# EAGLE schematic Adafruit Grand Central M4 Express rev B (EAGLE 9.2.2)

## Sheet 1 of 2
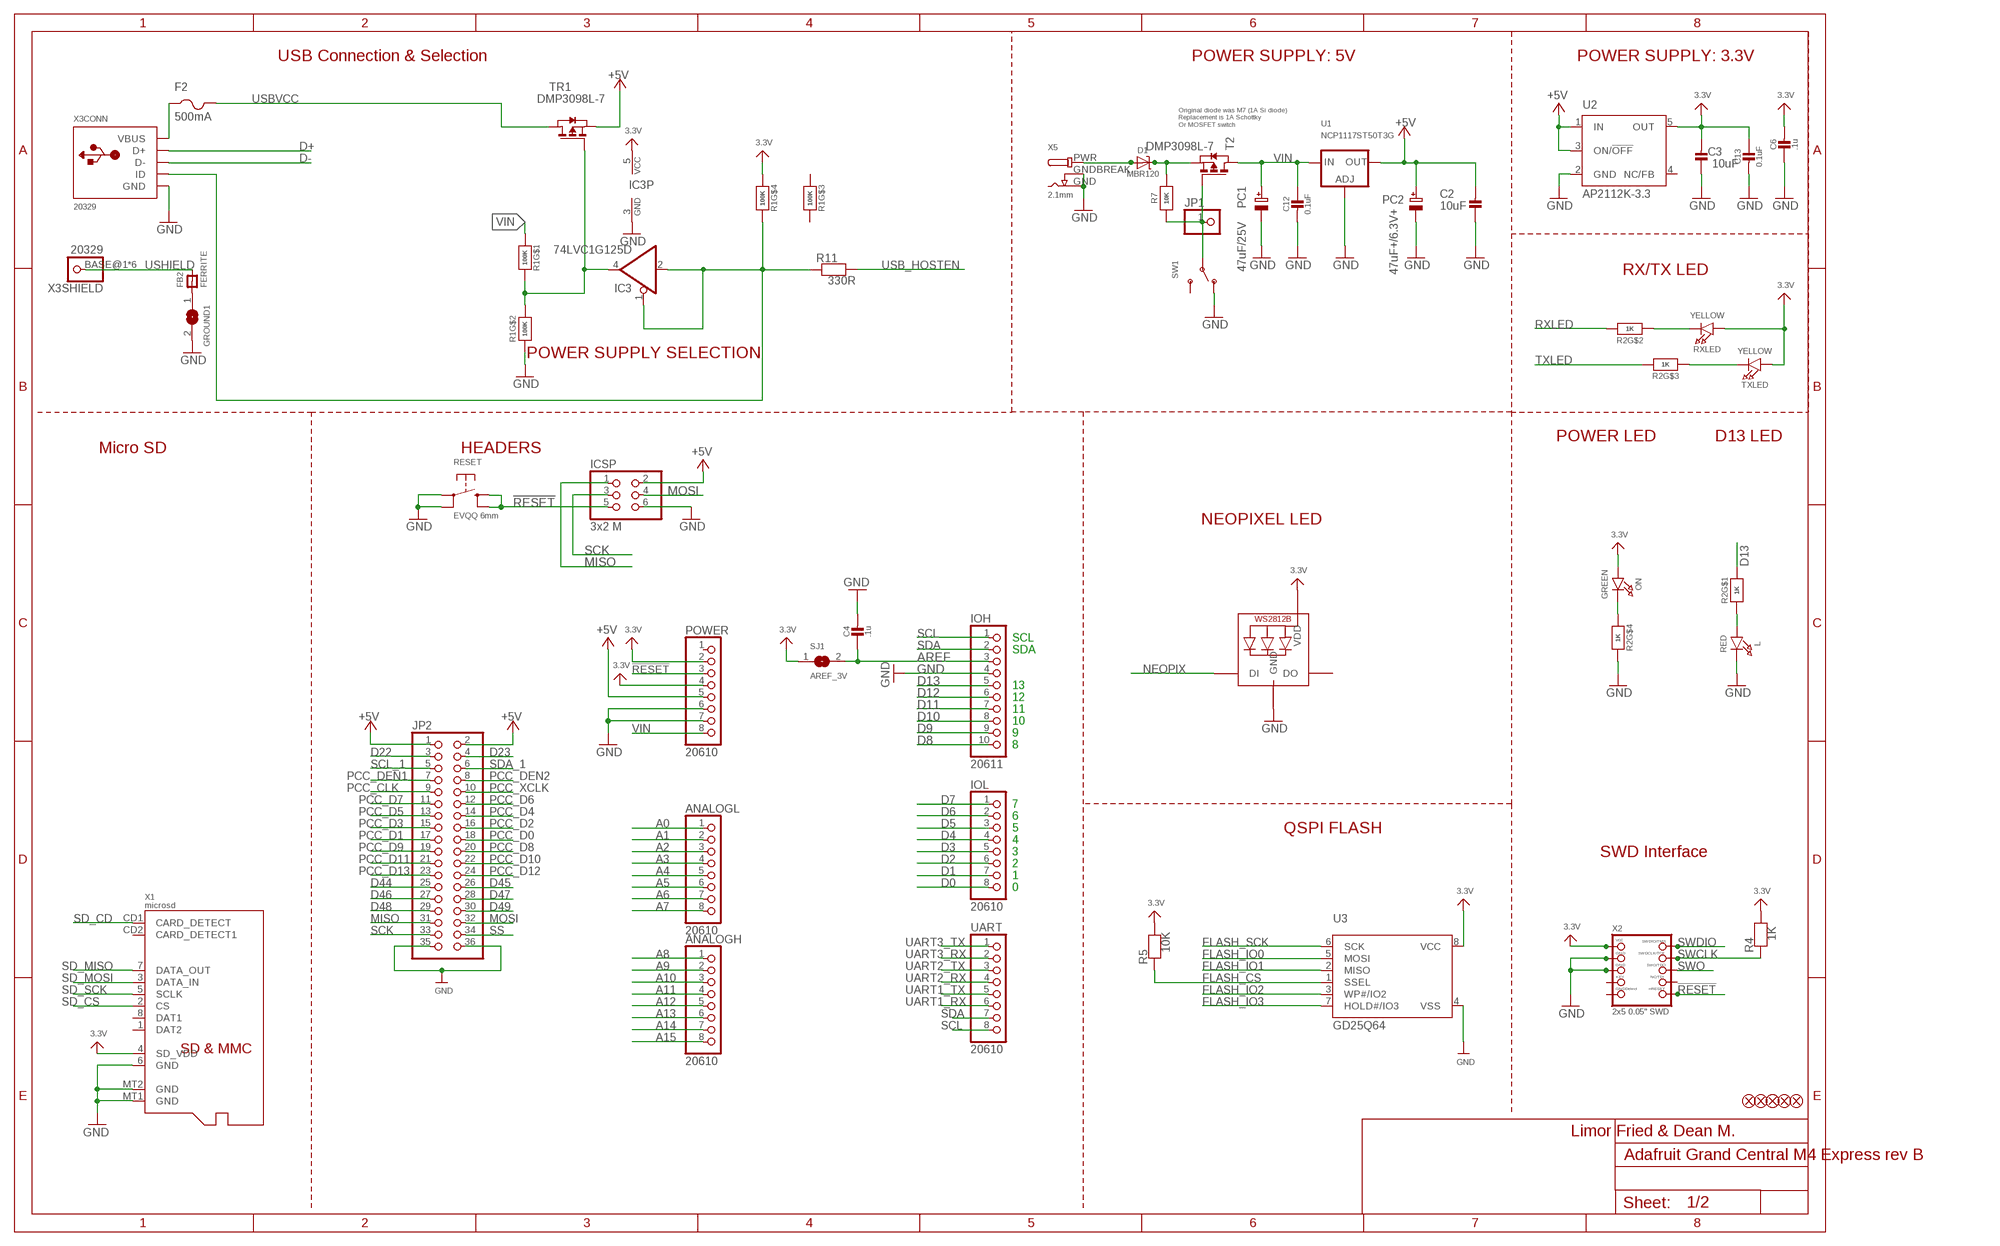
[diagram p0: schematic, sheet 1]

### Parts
ANALOGH  20610  HEADER-1X8OVALWAVE  [1X08_OVALWAVE]
ANALOGL  20610  HEADER-1X8OVALWAVE  [1X08_OVALWAVE]
C2  10uF  CAP_CERAMIC0805-NOOUTLINE  [0805-NO]
C3  10uF  CAP_CERAMIC0805-NOOUTLINE  [0805-NO]
C4  .1u  CAP_CERAMIC0603_NO  [0603-NO]
C6  .1u  CAP_CERAMIC0603_NO  [0603-NO]
C12  0.1uF  CAP_CERAMIC0603_NO  [0603-NO]
C13  0.1uF  CAP_CERAMIC0603_NO  [0603-NO]
D1  MBR120  DIODE-SCHOTTKYSOD-123  [SOD-123]
F2  500mA  PTCFUSE-1206  [R1206]
FB2  FERRITE  FERRITE-0805NO  [0805-NO]
FD1  FIDUCIAL_1MM  [FIDUCIAL_1MM]
FD2  FIDUCIAL_1MM  [FIDUCIAL_1MM]
FD3  FIDUCIAL_1MM  [FIDUCIAL_1MM]
FD4  FIDUCIAL_1MM  [FIDUCIAL_1MM]
FD5  FIDUCIAL_1MM  [FIDUCIAL_1MM]
GROUND1  SOLDERJUMPERCLOSED  [SOLDERJUMPER_CLOSEDWIRE]
IC3  74LVC1G125D  74AHC1G125DBV  [SOT23-5]
ICSP  3x2 M  HEADER-2X3  [2X03_ROUND_70MIL]
IOH  20611  HEADER-1X10OVALWAVE  [1X10_OVALWAVE]
IOL  20610  HEADER-1X8OVALWAVE  [1X08_OVALWAVE]
JP1  HEADER-1X1ROUND  [1X01_ROUND]
JP2  PINHD-2X18_THICKWAV  [2X18_THICKWAVE]
L  RED  LED0805_NOOUTLINE  [CHIPLED_0805_NOOUTLINE]
LED1  WS2812B3535  [LED3535]
ON  GREEN  LED0805_NOOUTLINE  [CHIPLED_0805_NOOUTLINE]
PC1  47uF/25V  CAP_ELECTROLYTICPANASONIC_D  [PANASONIC_D]
PC2  47uF+/6.3V+  CAP_ELECTROLYTICPANASONIC_D  [PANASONIC_D]
POWER  20610  HEADER-1X8OVALWAVE  [1X08_OVALWAVE]
R1  100K  RESISTOR_4PACK  [RESPACK_4X0603]
R2  1K  RESISTOR_4PACK  [RESPACK_4X0603]
R4  1K  RESISTOR_0603_NOOUT  [0603-NO]
R5  10K  RESISTOR_0603_NOOUT  [0603-NO]
R7  10K  RESISTOR_0603_NOOUT  [0603-NO]
R11  330R  RESISTOR_0603_NOOUT  [0603-NO]
RESET  EVQQ 6mm  SWITCH_TACT_SMT_EVQQ2_SMALL  [EVQ-Q2_SMALLER]
RXLED  YELLOW  LED0805_NOOUTLINE  [CHIPLED_0805_NOOUTLINE]
SJ1  AREF_3V  SOLDERJUMPERCLOSED  [SOLDERJUMPER_CLOSEDWIRE]
SW1  SWITCH_SPDT  [SPDT_SMT_SSSS811101]
T2  DMP3098L-7  PMOSSOT23  [SOT-23]
TR1  DMP3098L-7  0297_PMV48XP  [SOT-23]
TXLED  YELLOW  LED0805_NOOUTLINE  [CHIPLED_0805_NOOUTLINE]
U1  NCP1117ST50T3G  LM1117SOT223-REFLOW  [SOT223-R]
U2  AP2112K-3.3  LP2985-XXDBVR33  [SOT23-DBV]
U3  GD25Q64  SPIFLASH_SOIC8208MIL  [SOIC8_208MIL]
UART  20610  HEADER-1X8OVALWAVE  [1X08_OVALWAVE]
X1  microsd  MICROSD  [MICROSD]
X2  2x5 0.05" SWD  JTAG-CORTEXBOXPOSTS  [2X05_1.27MM_BOX_POSTS]
X3  20329  USB_W_SHIELD_V2  [4UCONN_20329_V2]
X5  2.1mm  DCBARRELPTH  [DCJACK_2MM_PTH]

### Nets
3.3V: C3.2 C6.2 C13.1 IC3.5(VCC) LED1.2(VDD) ON.A POWER.2 POWER.4 R1.4 R4.2 R5.2 RXLED.A SJ1.1 TXLED.A U2.5(OUT) U3.8(VCC) X1.4(SD_VDD) X2.1(VCC) ; also sheet 2
!RESET: ICSP.5 POWER.3 RESET.B'(S1) RESET.B(S) X2.10(NRESET) ; also sheet 2
+5V [usbvcc]: C2.2 ICSP.2 JP2.1 JP2.2 PC2.+ POWER.5 TR1.2(S) U1.2(OUT) U1.4(OUT) U2.1(IN) U2.3(ON/!OFF)
A0: ANALOGL.1 ; also sheet 2
A1: ANALOGL.2 ; also sheet 2
A2: ANALOGL.3 ; also sheet 2
A3: ANALOGL.4 ; also sheet 2
A4: ANALOGL.5 ; also sheet 2
A5: ANALOGL.6 ; also sheet 2
A6: ANALOGL.7 ; also sheet 2
A7: ANALOGL.8 ; also sheet 2
A8: ANALOGH.1 ; also sheet 2
A9: ANALOGH.2 ; also sheet 2
A10: ANALOGH.3 ; also sheet 2
A11: ANALOGH.4 ; also sheet 2
A12: ANALOGH.5 ; also sheet 2
A13: ANALOGH.6 ; also sheet 2
A14: ANALOGH.7 ; also sheet 2
A15: ANALOGH.8 ; also sheet 2
AREF [aref]: C4.1 IOH.3 SJ1.2 ; also sheet 2
D0: IOL.8 ; also sheet 2
D1: IOL.7 ; also sheet 2
D2: IOL.6 ; also sheet 2
D3: IOL.5 ; also sheet 2
D4: IOL.4 ; also sheet 2
D5: IOL.3 ; also sheet 2
D6: IOL.2 ; also sheet 2
D7: IOL.1 ; also sheet 2
D8: IOH.10 ; also sheet 2
D9: IOH.9 ; also sheet 2
D10: IOH.8 ; also sheet 2
D11: IOH.7 ; also sheet 2
D12: IOH.6 ; also sheet 2
D13: IOH.5 R2.8 ; also sheet 2
D22: JP2.3 ; also sheet 2
D23: JP2.4 ; also sheet 2
D44: JP2.25 ; also sheet 2
D45: JP2.26 ; also sheet 2
D46: JP2.27 ; also sheet 2
D47: JP2.28 ; also sheet 2
D48: JP2.29 ; also sheet 2
D49: JP2.30 ; also sheet 2
D+ [USB]: X3.D+(CONN:D+) ; also sheet 2
D- [USB]: X3.D-(CONN:D-) ; also sheet 2
FLASH_CS: R5.1 U3.1(SSEL) ; also sheet 2
FLASH_IO0: U3.5(MOSI) ; also sheet 2
FLASH_IO1: U3.2(MISO) ; also sheet 2
FLASH_IO2: U3.3(WP#/IO2) ; also sheet 2
FLASH_IO3: U3.7(HOLD#/IO3) ; also sheet 2
FLASH_SCK: U3.6(SCK) ; also sheet 2
GND [gnd]: C2.1 C3.1 C4.2 C6.1 C12.2 C13.2 GROUND1.2 IC3.3(GND) ICSP.6 IOH.4 JP2.35 JP2.36 L.C LED1.4(GND) PC1.- PC2.- POWER.6 POWER.7 R1.2 R2.5 RESET.A'(P1) RESET.A(P) SW1.A(O) U1.1(ADJ) U2.2(GND) U3.4(VSS) X1.6(GND) X1.MT1(GND) X1.MT2(GND) X2.3(GND) X2.5(GND) X3.GND(CONN:GND) X5.GND X5.GNDBREAK ; also sheet 2
MISO: ICSP.1 JP2.31 ; also sheet 2
MOSI: ICSP.4 JP2.32 ; also sheet 2
N$1: L.A R2.1
N$2: FB2.1 GROUND1.1
N$3: ON.C R2.4
N$5: R2.2 RXLED.C
N$7: R2.3 TXLED.C
N$10: IC3.1(OE) IC3.2(I) R1.5 R11.1 X3.ID(CONN:ID)
N$11: IC3.4(O) R1.7 R1.8 TR1.3(G)
N$15: D1.C R7.2 T2.2(S)
NEOPIX: LED1.1(DI) ; also sheet 2
PCC_CLK: JP2.9 ; also sheet 2
PCC_D0: JP2.18 ; also sheet 2
PCC_D1: JP2.17 ; also sheet 2
PCC_D2: JP2.16 ; also sheet 2
PCC_D3: JP2.15 ; also sheet 2
PCC_D4: JP2.14 ; also sheet 2
PCC_D5: JP2.13 ; also sheet 2
PCC_D6: JP2.12 ; also sheet 2
PCC_D7: JP2.11 ; also sheet 2
PCC_D8: JP2.20 ; also sheet 2
PCC_D9: JP2.19 ; also sheet 2
PCC_D10: JP2.22 ; also sheet 2
PCC_D11: JP2.21 ; also sheet 2
PCC_D12: JP2.24 ; also sheet 2
PCC_D13: JP2.23 ; also sheet 2
PCC_DEN1: JP2.7 ; also sheet 2
PCC_DEN2: JP2.8 ; also sheet 2
PCC_XCLK: JP2.10 ; also sheet 2
PWR_SWITCH: JP1.1 R7.1 SW1.B(P) T2.3(G)
PWRIN [USB]: D1.A X5.PWR
RXLED: R2.7 ; also sheet 2
SCK: ICSP.3 JP2.33 ; also sheet 2
SCL: IOH.1 UART.8 ; also sheet 2
SCL_1: JP2.5 ; also sheet 2
SD_CD: X1.CD1(CARD_DETECT) ; also sheet 2
SD_CS: X1.2(CS) ; also sheet 2
SD_MISO: X1.7(DATA_OUT) ; also sheet 2
SD_MOSI: X1.3(DATA_IN) ; also sheet 2
SD_SCK: X1.5(SCLK) ; also sheet 2
SDA: IOH.2 UART.7 ; also sheet 2
SDA_1: JP2.6 ; also sheet 2
SS: JP2.34 ; also sheet 2
SWCLK: R4.1 X2.4(SWDCLK) ; also sheet 2
SWDIO: X2.2(SWDIO) ; also sheet 2
SWO: X2.6(SWO) ; also sheet 2
TXLED: R2.6 ; also sheet 2
UART1_RX: UART.6 ; also sheet 2
UART1_TX: UART.5 ; also sheet 2
UART2_RX: UART.4 ; also sheet 2
UART2_TX: UART.3 ; also sheet 2
UART3_RX: UART.2 ; also sheet 2
UART3_TX: UART.1 ; also sheet 2
USB_HOSTEN: R11.2 ; also sheet 2
USBVCC [usbvcc]: F2.2 TR1.1(D)
USHIELD [gnd]: FB2.2 X3.BASE@1 X3.BASE@2 X3.SPRT@1 X3.SPRT@2 X3.SPRT@3 X3.SPRT@4
VBUS: F2.1 X3.VBUS(CONN:VBUS)
VIN [USB]: C12.1 PC1.+ POWER.8 R1.1 T2.1(D) U1.3(IN)
Unconnected: LED1.3(DO) POWER.1 R1.3 R1.6 SW1.C(S) U2.4(NC/FB) X1.1(DAT2) X1.8(DAT1) X1.CD2(CARD_DETECT1) X2.7(KEY) X2.8(TDI) X2.9(GNDDETECT)

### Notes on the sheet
- USB Connection & Selection | POWER SUPPLY: 5V | POWER SUPPLY: 3.3V
- Original diode was M7 (1A Si diode)
  Replacement is 1A Schottky
  Or MOSFET switch
- RX/TX LED
- POWER SUPPLY SELECTION
- POWER LED | D13 LED
- Micro SD | HEADERS
- NEOPIXEL LED
- SCL
- SDA
- 13
- 12
- 11
- 10
- 9
- 8
- 7
- 6
- 5 | QSPI FLASH
- 4
- 3 | SWD Interface
- 2
- 1
- 0
- Limor Fried & Dean M.

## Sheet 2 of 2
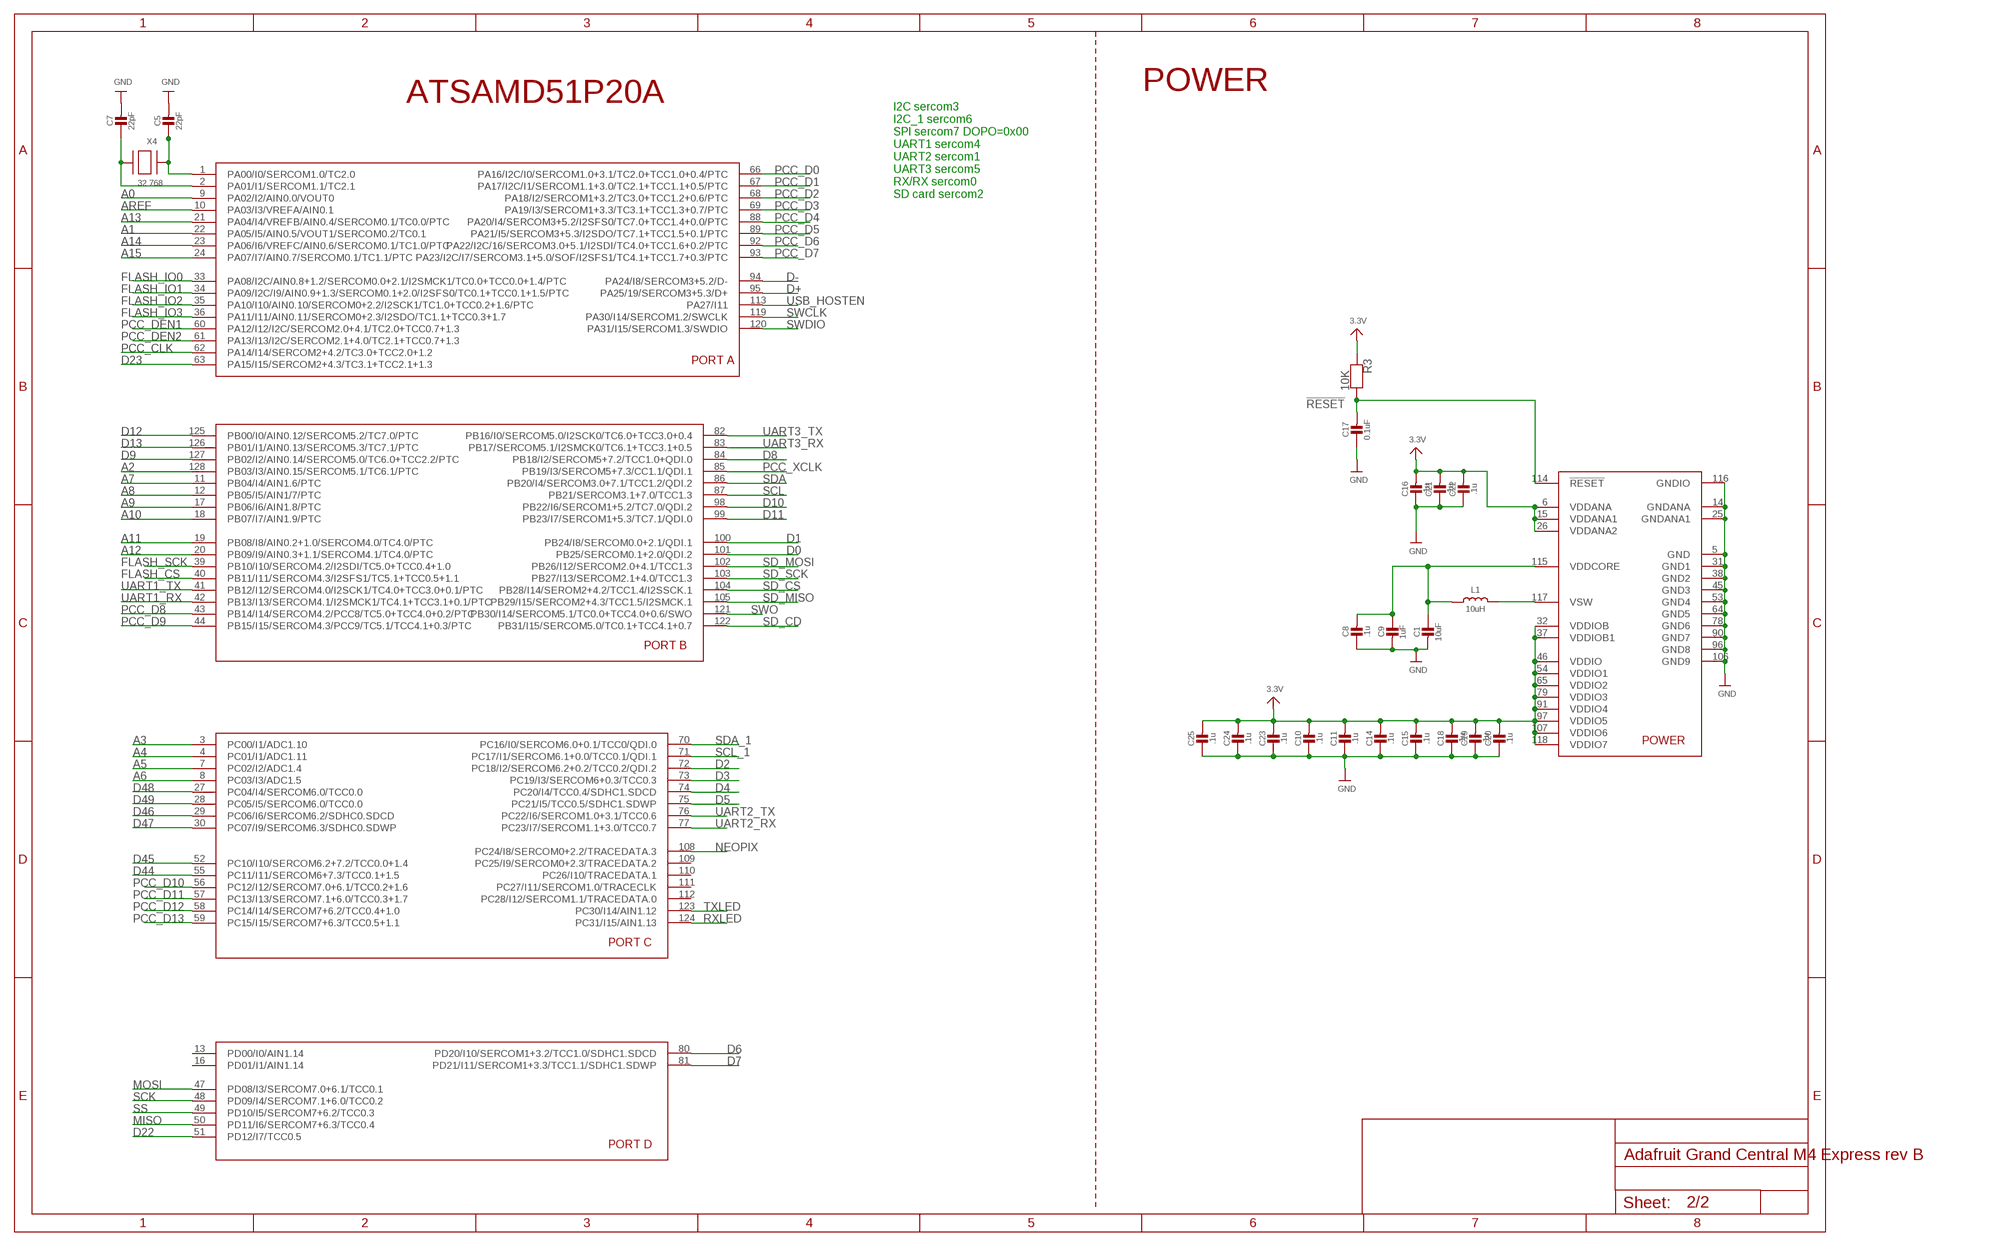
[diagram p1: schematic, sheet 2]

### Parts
C1  10uF  CAP_CERAMIC0805-NOOUTLINE  [0805-NO]
C5  22pF  CAP_CERAMIC0603_NO  [0603-NO]
C7  22pF  CAP_CERAMIC0603_NO  [0603-NO]
C8  .1u  CAP_CERAMIC0603_NO  [0603-NO]
C9  1uF  CAP_CERAMIC0603_NO  [0603-NO]
C10  .1u  CAP_CERAMIC0603_NO  [0603-NO]
C11  .1u  CAP_CERAMIC0603_NO  [0603-NO]
C14  .1u  CAP_CERAMIC0603_NO  [0603-NO]
C15  .1u  CAP_CERAMIC0603_NO  [0603-NO]
C16  .1u  CAP_CERAMIC0603_NO  [0603-NO]
C17  0.1uF  CAP_CERAMIC0603_NO  [0603-NO]
C18  .1u  CAP_CERAMIC0603_NO  [0603-NO]
C19  .1u  CAP_CERAMIC0603_NO  [0603-NO]
C20  .1u  CAP_CERAMIC0603_NO  [0603-NO]
C21  .1u  CAP_CERAMIC0603_NO  [0603-NO]
C22  .1u  CAP_CERAMIC0603_NO  [0603-NO]
C23  .1u  CAP_CERAMIC0603_NO  [0603-NO]
C24  .1u  CAP_CERAMIC0603_NO  [0603-NO]
C25  .1u  CAP_CERAMIC0603_NO  [0603-NO]
L1  10uH  INDUCTOR  [INDUCTOR_1007]
R3  10K  RESISTOR_0603_NOOUT  [0603-NO]
U$1  SAMD51PXXA  [SQFP-S-14X14-128]
X4  32.768  XTAL-3.2X1.5  [XTAL3215]

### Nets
3.3V: C10.2 C11.2 C14.2 C15.2 C16.2 C18.2 C19.2 C20.2 C21.2 C22.2 C23.2 C24.2 C25.2 R3.1 U$1.6(VDDANA) U$1.15(VDDANA1) U$1.26(VDDANA2) U$1.32(VDDIOB) U$1.37(VDDIOB1) U$1.46(VDDIO) U$1.54(VDDIO1) U$1.65(VDDIO2) U$1.79(VDDIO3) U$1.91(VDDIO4) U$1.97(VDDIO5) U$1.107(VDDIO6) U$1.118(VDDIO7) ; also sheet 1
!RESET: C17.2 R3.2 U$1.114(!RESET) ; also sheet 1
A0: U$1.9(PA02/I2/AIN0.0/VOUT0) ; also sheet 1
A1: U$1.22(PA05/I5/AIN0.5/VOUT1/SERCOM0.2/TC0.1) ; also sheet 1
A2: U$1.128(PB03/I3/AIN0.15/SERCOM5.1/TC6.1/PTC) ; also sheet 1
A3: U$1.3(PC00/I1/ADC1.10) ; also sheet 1
A4: U$1.4(PC01/I1/ADC1.11) ; also sheet 1
A5: U$1.7(PC02/I2/ADC1.4) ; also sheet 1
A6: U$1.8(PC03/I3/ADC1.5) ; also sheet 1
A7: U$1.11(PB04/I4/AIN1.6/PTC) ; also sheet 1
A8: U$1.12(PB05/I5/AIN1/7/PTC) ; also sheet 1
A9: U$1.17(PB06/I6/AIN1.8/PTC) ; also sheet 1
A10: U$1.18(PB07/I7/AIN1.9/PTC) ; also sheet 1
A11: U$1.19(PB08/I8/AIN0.2+1.0/SERCOM4.0/TC4.0/PTC) ; also sheet 1
A12: U$1.20(PB09/I9/AIN0.3+1.1/SERCOM4.1/TC4.0/PTC) ; also sheet 1
A13: U$1.21(PA04/I4/VREFB/AIN0.4/SERCOM0.1/TC0.0/PTC) ; also sheet 1
A14: U$1.23(PA06/I6/VREFC/AIN0.6/SERCOM0.1/TC1.0/PTC) ; also sheet 1
A15: U$1.24(PA07/I7/AIN0.7/SERCOM0.1/TC1.1/PTC) ; also sheet 1
AREF [aref]: U$1.10(PA03/I3/VREFA/AIN0.1) ; also sheet 1
D0: U$1.101(PB25/SERCOM0.1+2.0/QDI.2) ; also sheet 1
D1: U$1.100(PB24/I8/SERCOM0.0+2.1/QDI.1) ; also sheet 1
D2: U$1.72(PC18/I2/SERCOM6.2+0.2/TCC0.2/QDI.2) ; also sheet 1
D3: U$1.73(PC19/I3/SERCOM6+0.3/TCC0.3) ; also sheet 1
D4: U$1.74(PC20/I4/TCC0.4/SDHC1.SDCD) ; also sheet 1
D5: U$1.75(PC21/I5/TCC0.5/SDHC1.SDWP) ; also sheet 1
D6: U$1.80(PD20/I10/SERCOM1+3.2/TCC1.0/SDHC1.SDCD) ; also sheet 1
D7: U$1.81(PD21/I11/SERCOM1+3.3/TCC1.1/SDHC1.SDWP) ; also sheet 1
D8: U$1.84(PB18/I2/SERCOM5+7.2/TCC1.0+QDI.0) ; also sheet 1
D9: U$1.127(PB02/I2/AIN0.14/SERCOM5.0/TC6.0+TCC2.2/PTC) ; also sheet 1
D10: U$1.98(PB22/I6/SERCOM1+5.2/TC7.0/QDI.2) ; also sheet 1
D11: U$1.99(PB23/I7/SERCOM1+5.3/TC7.1/QDI.0) ; also sheet 1
D12: U$1.125(PB00/I0/AIN0.12/SERCOM5.2/TC7.0/PTC) ; also sheet 1
D13: U$1.126(PB01/I1/AIN0.13/SERCOM5.3/TC7.1/PTC) ; also sheet 1
D22: U$1.51(PD12/I7/TCC0.5) ; also sheet 1
D23: U$1.63(PA15/I15/SERCOM2+4.3/TC3.1+TCC2.1+1.3) ; also sheet 1
D44: U$1.55(PC11/I11/SERCOM6+7.3/TCC0.1+1.5) ; also sheet 1
D45: U$1.52(PC10/I10/SERCOM6.2+7.2/TCC0.0+1.4) ; also sheet 1
D46: U$1.29(PC06/I6/SERCOM6.2/SDHC0.SDCD) ; also sheet 1
D47: U$1.30(PC07/I9/SERCOM6.3/SDHC0.SDWP) ; also sheet 1
D48: U$1.27(PC04/I4/SERCOM6.0/TCC0.0) ; also sheet 1
D49: U$1.28(PC05/I5/SERCOM6.0/TCC0.0) ; also sheet 1
D+ [USB]: U$1.95(PA25/19/SERCOM3+5.3/D+) ; also sheet 1
D- [USB]: U$1.94(PA24/I8/SERCOM3+5.2/D-) ; also sheet 1
FLASH_CS: U$1.40(PB11/I11/SERCOM4.3/I2SFS1/TC5.1+TCC0.5+1.1) ; also sheet 1
FLASH_IO0: U$1.33(PA08/I2C/AIN0.8+1.2/SERCOM0.0+2.1/I2SMCK1/TC0.0+TCC0.0+1.4/PTC) ; also sheet 1
FLASH_IO1: U$1.34(PA09/I2C/I9/AIN0.9+1.3/SERCOM0.1+2.0/I2SFS0/TC0.1+TCC0.1+1.5/PTC) ; also sheet 1
FLASH_IO2: U$1.35(PA10/I10/AIN0.10/SERCOM0+2.2/I2SCK1/TC1.0+TCC0.2+1.6/PTC) ; also sheet 1
FLASH_IO3: U$1.36(PA11/I11/AIN0.11/SERCOM0+2.3/I2SDO/TC1.1+TCC0.3+1.7) ; also sheet 1
FLASH_SCK: U$1.39(PB10/I10/SERCOM4.2/I2SDI/TC5.0+TCC0.4+1.0) ; also sheet 1
GND [gnd]: C1.2 C5.2 C7.2 C8.1 C9.2 C10.1 C11.1 C14.1 C15.1 C16.1 C17.1 C18.1 C19.1 C20.1 C21.1 C22.1 C23.1 C24.1 C25.1 U$1.5(GND) U$1.14(GNDANA) U$1.25(GNDANA1) U$1.31(GND1) U$1.38(GND2) U$1.45(GND3) U$1.53(GND4) U$1.64(GND5) U$1.78(GND6) U$1.90(GND7) U$1.96(GND8) U$1.106(GND9) U$1.116(GNDIO) ; also sheet 1
MISO: U$1.50(PD11/I6/SERCOM7+6.3/TCC0.4) ; also sheet 1
MOSI: U$1.47(PD08/I3/SERCOM7.0+6.1/TCC0.1) ; also sheet 1
N$4: L1.P$2 U$1.117(VSW)
N$9: C5.1 U$1.1(PA00/I0/SERCOM1.0/TC2.0) X4.P$1
N$12: C7.1 U$1.2(PA01/I1/SERCOM1.1/TC2.1) X4.P$2
NEOPIX: U$1.108(PC24/I8/SERCOM0+2.2/TRACEDATA.3) ; also sheet 1
PCC_CLK: U$1.62(PA14/I14/SERCOM2+4.2/TC3.0+TCC2.0+1.2) ; also sheet 1
PCC_D0: U$1.66(PA16/I2C/I0/SERCOM1.0+3.1/TC2.0+TCC1.0+0.4/PTC) ; also sheet 1
PCC_D1: U$1.67(PA17/I2C/I1/SERCOM1.1+3.0/TC2.1+TCC1.1+0.5/PTC) ; also sheet 1
PCC_D2: U$1.68(PA18/I2/SERCOM1+3.2/TC3.0+TCC1.2+0.6/PTC) ; also sheet 1
PCC_D3: U$1.69(PA19/I3/SERCOM1+3.3/TC3.1+TCC1.3+0.7/PTC) ; also sheet 1
PCC_D4: U$1.88(PA20/I4/SERCOM3+5.2/I2SFS0/TC7.0+TCC1.4+0.0/PTC) ; also sheet 1
PCC_D5: U$1.89(PA21/I5/SERCOM3+5.3/I2SDO/TC7.1+TCC1.5+0.1/PTC) ; also sheet 1
PCC_D6: U$1.92(PA22/I2C/16/SERCOM3.0+5.1/I2SDI/TC4.0+TCC1.6+0.2/PTC) ; also sheet 1
PCC_D7: U$1.93(PA23/I2C/I7/SERCOM3.1+5.0/SOF/I2SFS1/TC4.1+TCC1.7+0.3/PTC) ; also sheet 1
PCC_D8: U$1.43(PB14/I14/SERCOM4.2/PCC8/TC5.0+TCC4.0+0.2/PTC) ; also sheet 1
PCC_D9: U$1.44(PB15/I15/SERCOM4.3/PCC9/TC5.1/TCC4.1+0.3/PTC) ; also sheet 1
PCC_D10: U$1.56(PC12/I12/SERCOM7.0+6.1/TCC0.2+1.6) ; also sheet 1
PCC_D11: U$1.57(PC13/I13/SERCOM7.1+6.0/TCC0.3+1.7) ; also sheet 1
PCC_D12: U$1.58(PC14/I14/SERCOM7+6.2/TCC0.4+1.0) ; also sheet 1
PCC_D13: U$1.59(PC15/I15/SERCOM7+6.3/TCC0.5+1.1) ; also sheet 1
PCC_DEN1: U$1.60(PA12/I12/I2C/SERCOM2.0+4.1/TC2.0+TCC0.7+1.3) ; also sheet 1
PCC_DEN2: U$1.61(PA13/I13/I2C/SERCOM2.1+4.0/TC2.1+TCC0.7+1.3) ; also sheet 1
PCC_XCLK: U$1.85(PB19/I3/SERCOM5+7.3/CC1.1/QDI.1) ; also sheet 1
RXLED: U$1.124(PC31/I15/AIN1.13) ; also sheet 1
SCK: U$1.48(PD09/I4/SERCOM7.1+6.0/TCC0.2) ; also sheet 1
SCL: U$1.87(PB21/SERCOM3.1+7.0/TCC1.3) ; also sheet 1
SCL_1: U$1.71(PC17/I1/SERCOM6.1+0.0/TCC0.1/QDI.1) ; also sheet 1
SD_CD: U$1.122(PB31/I15/SERCOM5.0/TC0.1+TCC4.1+0.7) ; also sheet 1
SD_CS: U$1.104(PB28/I14/SEROM2+4.2/TCC1.4/I2SSCK.1) ; also sheet 1
SD_MISO: U$1.105(PB29/I15/SERCOM2+4.3/TCC1.5/I2SMCK.1) ; also sheet 1
SD_MOSI: U$1.102(PB26/I12/SERCOM2.0+4.1/TCC1.3) ; also sheet 1
SD_SCK: U$1.103(PB27/I13/SERCOM2.1+4.0/TCC1.3) ; also sheet 1
SDA: U$1.86(PB20/I4/SERCOM3.0+7.1/TCC1.2/QDI.2) ; also sheet 1
SDA_1: U$1.70(PC16/I0/SERCOM6.0+0.1/TCC0/QDI.0) ; also sheet 1
SS: U$1.49(PD10/I5/SERCOM7+6.2/TCC0.3) ; also sheet 1
SWCLK: U$1.119(PA30/I14/SERCOM1.2/SWCLK) ; also sheet 1
SWDIO: U$1.120(PA31/I15/SERCOM1.3/SWDIO) ; also sheet 1
SWO: U$1.121(PB30/I14/SERCOM5.1/TC0.0+TCC4.0+0.6/SWO) ; also sheet 1
TXLED: U$1.123(PC30/I14/AIN1.12) ; also sheet 1
UART1_RX: U$1.42(PB13/I13/SERCOM4.1/I2SMCK1/TC4.1+TCC3.1+0.1/PTC) ; also sheet 1
UART1_TX: U$1.41(PB12/I12/SERCOM4.0/I2SCK1/TC4.0+TCC3.0+0.1/PTC) ; also sheet 1
UART2_RX: U$1.77(PC23/I7/SERCOM1.1+3.0/TCC0.7) ; also sheet 1
UART2_TX: U$1.76(PC22/I6/SERCOM1.0+3.1/TCC0.6) ; also sheet 1
UART3_RX: U$1.83(PB17/SERCOM5.1/I2SMCK0/TC6.1+TCC3.1+0.5) ; also sheet 1
UART3_TX: U$1.82(PB16/I0/SERCOM5.0/I2SCK0/TC6.0+TCC3.0+0.4) ; also sheet 1
USB_HOSTEN: U$1.113(PA27/I11) ; also sheet 1
VDDCORE: C1.1 C8.2 C9.1 L1.P$1 U$1.115(VDDCORE)
Unconnected: U$1.13(PD00/I0/AIN1.14) U$1.16(PD01/I1/AIN1.14) U$1.109(PC25/I9/SERCOM0+2.3/TRACEDATA.2) U$1.110(PC26/I10/TRACEDATA.1) U$1.111(PC27/I11/SERCOM1.0/TRACECLK) U$1.112(PC28/I12/SERCOM1.1/TRACEDATA.0)

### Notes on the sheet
- POWER
- ATSAMD51P20A
- I2C sercom3
  I2C_1 sercom6
  SPI sercom7 DOPO=0x00
  UART1 sercom4
  UART2 sercom1
  UART3 sercom5
  RX/RX sercom0
  SD card sercom2

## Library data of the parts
ANALOGH ANALOGL IOL POWER UART = microbuilder:HEADER-1X8: PIN HEADER
C1-C25 = microbuilder:CAP_CERAMIC: Ceramic Capacitors
D1 = microbuilder:DIODE-SCHOTTKY
F2 = adafruit:PTCFUSE: PTC fuses, resettable thermistors
FB2 = microbuilder:FERRITE: Ferrite Bead
FD1-FD5 = microbuilder:FIDUCIAL: Fiducial Alignment Points; BOM: EXCLUDE
GROUND1 SJ1 = microbuilder:SOLDERJUMPER: SMD Solder JUMPER
IC3 = 74xx-little-de:74*1G125: Single Bus Buffer Gate with 3-State Output
ICSP = microbuilder:HEADER-2X3: PIN HEADER
IOH = microbuilder:HEADER-1X10: PIN HEADER
JP1 = microbuilder:HEADER-1X1: PIN HEADER
JP2 = microbuilder:PINHD-2X18: PIN HEADER
L ON RXLED TXLED = microbuilder:LED: LED
L1 = microbuilder:INDUCTOR: Inductors
LED1 = microbuilder:WS2812B
PC1 PC2 = microbuilder:CAP_ELECTROLYTIC: Electrolytic Capacitors
R1 R2 = microbuilder:RESISTOR_4PACK: Resistor Packs (4 resistors) 4 x 0603 10K 1/16W - Digikey: YC164J-10KCT-ND
R3-R5 R7 R11 = microbuilder:RESISTOR: Resistors
RESET = microbuilder:SWITCH_TACT_SMT: SMT Tact Switches 6x6mm - Digikey: P12940SCT-ND KMR2 (4.6x2.8mm) - Digikey: 401-1426-1-ND EVQ-PQHB55 - Light Touch, 160GF (4.5x4.5mm) - Digikey: P8090SCT-ND KMT0 - KMT021 NGJ LHS (etc.) IP68/Waterproof - Digikey: CKN10289CT-ND
SW1 = microbuilder:SWITCH_SPDT: Switch - SPDT SSSS811101 - Horizontal Two Position SMT, 0.3A 4V [Mouser: 688-SSSS811101]
T2 = zetex:PMOSSOT23: MOS FET; OC_FARNELL: unknown; OC_NEWARK: unknown
TR1 = Transistors:0297_PMV48XP: 20 V, 3.5 A P-channel Trench MOSFET - PMV48XP; CASE: SOT23; MONTHLY_USAGE: _____; PART_NUMBER: PMV48XP; PRICE: _____; SUPPLIER: _____; TYPE: Transistor; VALUE: PMV48XP
U1 = microbuilder:LM1117: LM1117 Voltage Regulator LM1117 Adjustable Voltage regulator [Digikey: LM1117IMP-ADJDKR-ND] LM1117 3.3V Voltage regulator [AP1117E33GDIDKR-ND] LM1117 5.0V Voltage regulator [AP1117E50GDIDKR-ND] SOT223-REFLOW - SOT223 package for solder paste/reflow ovens SOT223-WAVE - SOT223 package for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
U2 = SmartPrj:LP2985-XXDBVR: ULTRALOW-POWER 50-mA LOW-DROPOUT LINEAR REGULATORS 50-mA Low-Dropout Regulator Source: http://focus.ti.com/lit/ds/symlink/tps77001.pdf
U3 = microbuilder:SPIFLASH_SOIC8: SOIC8 SPI Flash Be careful with the size since SOIC8 flash comes in several 'widths' SOIC8 150 mil M25P16 - 16Mbit (2Mbit x 8) Serial Flash (75MHz SPI Bus), Supply: 2.7-3.6V Digikey: SOIC8 - M25P16-VMN6P-ND SOIC8 208 mil W25Q16BVSSIG - 16Mbit (2Mbit x 8) Serial Flash (104MHz SPI Bus), Supply: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
U$1 = microbuilder:SAMD51PXXA: SAMD51 P variant
X1 = microbuilder:MICROSD: MicroSD/Transflash Card Holder with SPI pinout 3M: 2908-05WB-MG 4UConnector: 19656 Footprint courtesy: Adafruit Industries
X2 = microbuilder:JTAG-CORTEX: Serial Wire (SW-DP) Connector Standard 0.05" 10-pin connector is for use with the Cortex M and Cortex A SWD (serial wire debugger) interface (SW-DP) Connectors 2x05_1.27MM_SMT - Inexpensive surface-mount header with bare pins, compatible with standard 10-pin SWD cables (4UCON: 16846)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
X3 = microbuilder:USB_W_SHIELD
X4 = adafruit2:XTAL: Low cost SMT crystals, no capacitors included
X5 = microbuilder:DCBARREL: DC Barrel Jack DCJACK_1.3MM_PTH - Through Hole 1.3mm Jack (4UConnector: 05536) DCJACK_2MM_PTH - Through Hole 2.0/2.1 Jack (4UConnector: 05537) DCJACK_2MM_SMT - SMT 2.0/2.1mm Jack(4UConnector: 03267)

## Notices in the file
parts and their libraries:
microbuilder: This work is placed in the public domain, and may be freely used for commercial and non-commercial work with the following conditions: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
